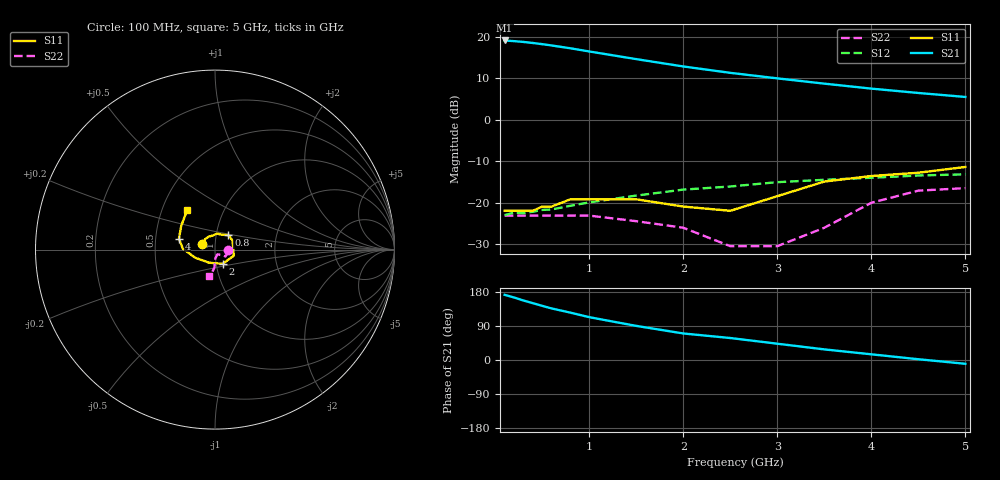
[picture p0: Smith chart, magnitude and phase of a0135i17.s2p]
!  MSA-0135 S AND NOISE PARAMETERS
!  Id=17mA  LAST UPDATED 07-22-92
# ghz s ma r 50
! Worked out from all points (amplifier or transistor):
!   16 points, 100 MHz to 5 GHz, reference 50 ohm
!   highest |S21| = 19.1 dB at 100 MHz (marker M1)
!   |S21| within 3 dB of that: start of sweep to 1.095 GHz
!   unconditionally stable (mu >= 1): start of sweep to end of sweep
!   at 300 MHz: K = 1.08, MAG = 18.9 dB, |S12| = -22.5 dB
!   at 1.5 GHz: K = 1.09, MAG = 14.7 dB, |S12| = -18.3 dB
!   at 5 GHz: K = 1.27, MAG = 6.2 dB, |S12| = -13.2 dB
!   lowest NFmin = 5.20 dB at 100 MHz
!   S11 on the Smith chart (normalised r, x): 100 MHz: 0.86, +0.05; 800 MHz: 1.15, +0.19; 2 GHz: 1.07, -0.17; 4 GHz: 0.66, +0.08; 5 GHz: 0.67, +0.32
0.1  0.08 158.0  9.01 172.0  0.071 3.0  0.07 -2.0
0.2  0.08 134.0  8.84 165.0  0.076 6.0  0.07 -10.0
0.3  0.08 116.0  8.65 157.0  0.075 12.0  0.07 -10.0
0.4  0.08 97.0  8.4 150.0  0.078 13.0  0.07 -15.0
0.5  0.09 83.0  8.13 143.0  0.082 16.0  0.07 -17.0
0.6  0.09 68.0  7.84 136.0  0.083 17.0  0.07 -21.0
0.8  0.11 47.0  7.25 125.0  0.092 22.0  0.07 -30.0
1  0.11 27.0  6.64 113.0  0.101 23.0  0.07 -34.0
1.5  0.11 -18.0  5.37 90.0  0.122 27.0  0.06 -34.0
2  0.09 -62.0  4.38 70.0  0.144 24.0  0.05 -39.0
2.5  0.08 -114.0  3.67 58.0  0.157 24.0  0.03 -61.0
3  0.12 -158.0  3.15 43.0  0.177 20.0  0.03 -67.0
3.5  0.18 178.0  2.72 28.0  0.189 14.0  0.05 -88.0
4  0.21 163.0  2.37 15.0  0.2 9.0  0.1 -92.0
4.5  0.23 145.0  2.1 2.0  0.213 4.0  0.14 -99.0
5  0.27 125.0  1.88 -10.0  0.22 -2.0  0.15 -102.0
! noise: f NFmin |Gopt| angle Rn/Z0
0.1  5.2  0.23  1  1.13
0.5  5.3  0.23  5  1.13
1  5.5  0.21  9  1.11
2  5.8  0.18  17  1.1
